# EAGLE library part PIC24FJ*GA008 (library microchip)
64/80/100-Pin General Purpose, 16-Bit Flash Microcontrollers Source: http://ww1.microchip.com/downloads/en/DeviceDoc/39747d.pdf
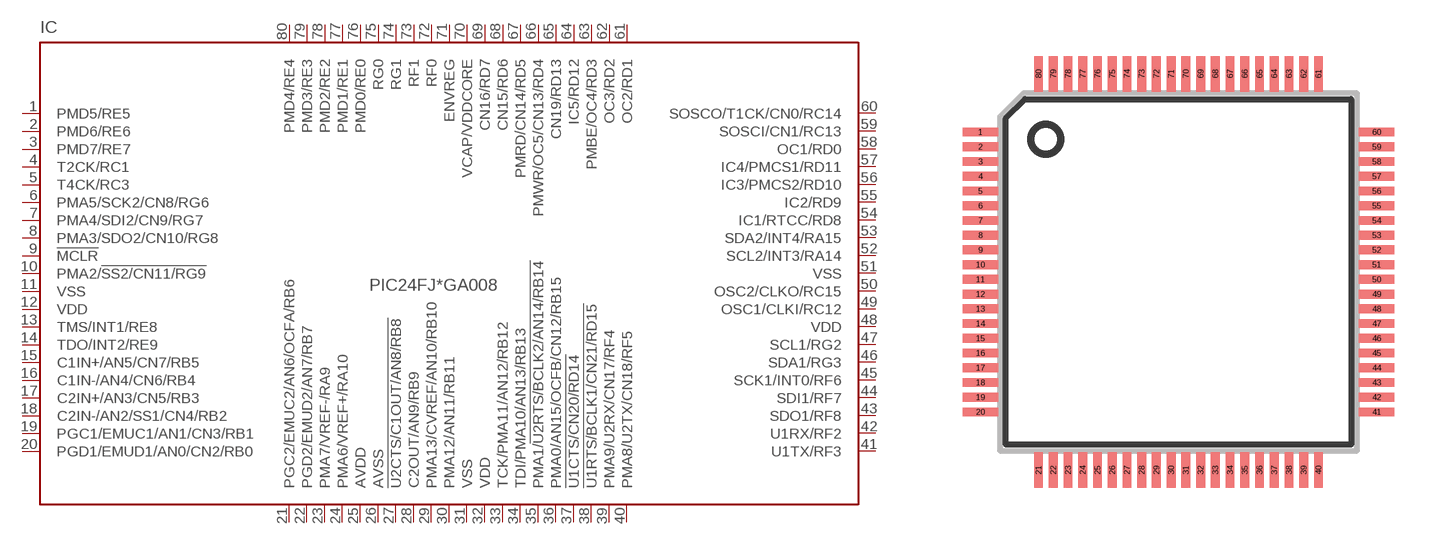
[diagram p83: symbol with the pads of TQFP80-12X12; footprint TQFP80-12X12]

Designator prefix IC

## PIC24FJ128GA008 (MF: MICROCHIP; MPN: PIC24FJ128GA008-I/PT; OC_FARNELL: 1146521; OC_NEWARK: 56K7339), PIC24FJ64GA008 (MPN: PIC24FJ64GA008-I/PT; OC_FARNELL: 1146525; OC_NEWARK: 56K7345), PIC24FJ96GA008 (MPN: PIC24FJ96GA008-I/PT; OC_FARNELL: 1146529; OC_NEWARK: 56K7351)  [TQFP80-12X12]
1  PMD5/RE5
2  PMD6/RE6
3  PMD7/RE7
4  T2CK/RC1
5  T4CK/RC3
6  PMA5/SCK2/CN8/RG6
7  PMA4/SDI2/CN9/RG7
8  PMA3/SDO2/CN10/RG8
9  !MCLR
10  PMA2/!SS2/CN11/RG9
11  VSS  pwr
12  VDD  pwr
13  TMS/INT1/RE8
14  TDO/INT2/RE9
15  C1IN+/AN5/CN7/RB5
16  C1IN-/AN4/CN6/RB4
17  C2IN+/AN3/CN5/RB3
18  C2IN-/AN2/SS1/CN4/RB2
19  PGC1/EMUC1/AN1/CN3/RB1
20  PGD1/EMUD1/AN0/CN2/RB0
21  PGC2/EMUC2/AN6/OCFA/RB6
22  PGD2/EMUD2/AN7/RB7
23  PMA7/VREF-/RA9
24  PMA6/VREF+/RA10
25  AVDD  pwr
26  AVSS  pwr
27  !U2CTS/C1OUT/AN8/RB8
28  C2OUT/AN9/RB9
29  PMA13/CVREF/AN10/RB10
30  PMA12/AN11/RB11
31  VSS  pwr
32  VDD  pwr
33  TCK/PMA11/AN12/RB12
34  TDI/PMA10/AN13/RB13
35  PMA1/!U2RTS/BCLK2/AN14/RB14
36  PMA0/AN15/OCFB/CN12/RB15
37  !U1CTS/CN20/RD14
38  !U1RTS/BCLK1/CN21/RD15
39  PMA9/U2RX/CN17/RF4
40  PMA8/U2TX/CN18/RF5
41  U1TX/RF3
42  U1RX/RF2
43  SDO1/RF8
44  SDI1/RF7
45  SCK1/INT0/RF6
46  SDA1/RG3
47  SCL1/RG2
48  VDD  pwr
49  OSC1/CLKI/RC12
50  OSC2/CLKO/RC15
51  VSS  pwr
52  SCL2/INT3/RA14
53  SDA2/INT4/RA15
54  IC1/RTCC/RD8
55  IC2/RD9
56  IC3/PMCS2/RD10
57  IC4/PMCS1/RD11
58  OC1/RD0
59  SOSCI/CN1/RC13
60  SOSCO/T1CK/CN0/RC14
61  OC2/RD1
62  OC3/RD2
63  PMBE/OC4/RD3
64  IC5/RD12
65  CN19/RD13
66  PMWR/OC5/CN13/RD4
67  PMRD/CN14/RD5
68  CN15/RD6
69  CN16/RD7
70  VCAP/VDDCORE
71  ENVREG
72  RF0
73  RF1
74  RG1
75  RG0
76  PMD0/RE0
77  PMD1/RE1
78  PMD2/RE2
79  PMD3/RE3
80  PMD4/RE4

## Footprint TQFP80-12X12 (pad centres in mm)
TQFP80 12x12x1 mm Body Source: http://www.microchip.com/ .. 39663c.pdf
smd 1.2 x 0.3: 1 -6.725,4.75; 2 -6.725,4.25; 3 -6.725,3.75; 4 -6.725,3.25; 5 -6.725,2.75; 6 -6.725,2.25; 7 -6.725,1.75; 8 -6.725,1.25; 9 -6.725,0.75; 10 -6.725,0.25; 11 -6.725,-0.25; 12 -6.725,-0.75; 13 -6.725,-1.25; 14 -6.725,-1.75; 15 -6.725,-2.25; 16 -6.725,-2.75; 17 -6.725,-3.25; 18 -6.725,-3.75; 19 -6.725,-4.25; 20 -6.725,-4.75; 41 6.725,-4.75; 42 6.725,-4.25; 43 6.725,-3.75; 44 6.725,-3.25; 45 6.725,-2.75; 46 6.725,-2.25; 47 6.725,-1.75; 48 6.725,-1.25; 49 6.725,-0.75; 50 6.725,-0.25; 51 6.725,0.25; 52 6.725,0.75; 53 6.725,1.25; 54 6.725,1.75; 55 6.725,2.25; 56 6.725,2.75; 57 6.725,3.25; 58 6.725,3.75; 59 6.725,4.25; 60 6.725,4.75
smd 0.3 x 1.2: 21 -4.75,-6.725; 22 -4.25,-6.725; 23 -3.75,-6.725; 24 -3.25,-6.725; 25 -2.75,-6.725; 26 -2.25,-6.725; 27 -1.75,-6.725; 28 -1.25,-6.725; 29 -0.75,-6.725; 30 -0.25,-6.725; 31 0.25,-6.725; 32 0.75,-6.725; 33 1.25,-6.725; 34 1.75,-6.725; 35 2.25,-6.725; 36 2.75,-6.725; 37 3.25,-6.725; 38 3.75,-6.725; 39 4.25,-6.725; 40 4.75,-6.725; 61 4.75,6.725; 62 4.25,6.725; 63 3.75,6.725; 64 3.25,6.725; 65 2.75,6.725; 66 2.25,6.725; 67 1.75,6.725; 68 1.25,6.725; 69 0.75,6.725; 70 0.25,6.725; 71 -0.25,6.725; 72 -0.75,6.725; 73 -1.25,6.725; 74 -1.75,6.725; 75 -2.25,6.725; 76 -2.75,6.725; 77 -3.25,6.725; 78 -3.75,6.725; 79 -4.25,6.725; 80 -4.75,6.725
